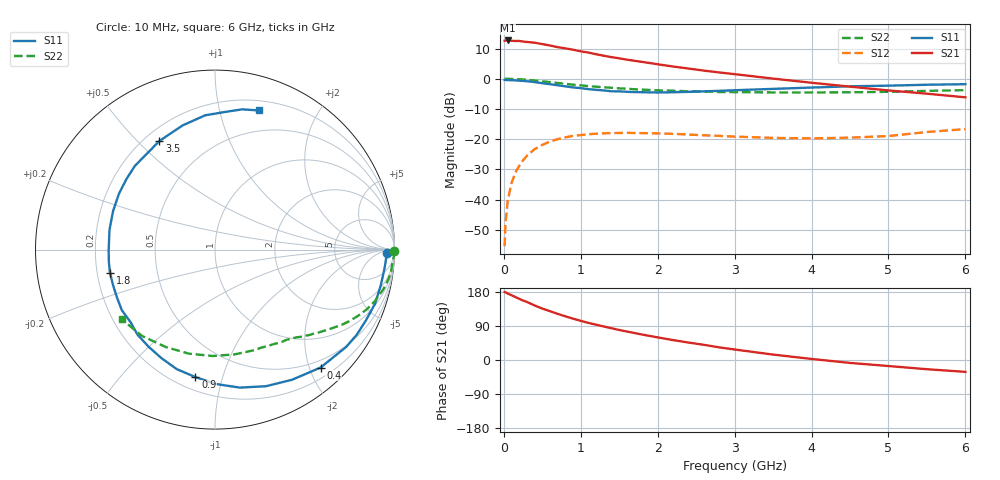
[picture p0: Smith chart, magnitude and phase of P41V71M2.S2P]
! SIEMENS Small Signal Semiconductors
! BFP182
! Si NPN RF Bipolar Junction Transistor in SOT143
! VCE = 1.75 V  IC = 1.2 mA
! Common Emitter S-Parameters:  March  1996
# GHz  S  MA  R  50
!  f  S11  S21  S12  S22
! GHz  MAG  ANG  MAG  ANG  MAG  ANG  MAG  ANG
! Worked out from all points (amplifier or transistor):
!   36 points, 10 MHz to 6 GHz, reference 50 ohm
!   highest |S21| = 12.7 dB at 50 MHz (marker M1)
!   |S21| within 3 dB of that: start of sweep to 884.8 MHz
!   unconditionally stable (mu >= 1): 2.497 GHz to end of sweep
!   at 250 MHz: K = 0.10, MSG = 19.6 dB, |S12| = -27.0 dB
!   at 1.4 GHz: K = 0.58, MSG = 12.6 dB, |S12| = -18.0 dB
!   at 6 GHz: K = 1.07, MAG = 3.6 dB, |S12| = -16.7 dB
!   S11 on the Smith chart (normalised r, x): 10 MHz: 37, -16; 400 MHz: 0.37, -2.18; 900 MHz: 0.28, -0.82; 1.8 GHz: 0.25, -0.10; 3.5 GHz: 0.26, +0.58; 6 GHz: 0.29, +1.32
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0.01  0.9558 -1.1  4.259 179.4  0.0017 88.1  0.9985 -0.4
0.02  0.9552 -2.6  4.273 178.8  0.0038 81.7  0.9999 -1.0
0.05  0.9505 -6.3  4.3 175.4  0.0096 89.3  0.9966 -2.3
0.1  0.9447 -12.2  4.251 170.9  0.0188 82.2  0.9905 -4.7
0.15  0.9413 -18.6  4.211 166.2  0.028 78.3  0.9889 -7.1
0.2  0.929 -25.0  4.221 161.4  0.0362 74.7  0.981 -9.4
0.4  0.8819 -48.2  3.947 143.9  0.0684 61.1  0.9365 -17.8
0.5  0.8426 -59.4  3.745 135.8  0.0805 54.5  0.9077 -21.6
0.6  0.8122 -69.6  3.55 128.7  0.0915 48.7  0.8785 -24.8
0.7  0.7813 -79.8  3.329 121.8  0.1002 43.6  0.8513 -27.7
0.8  0.7492 -89.4  3.183 115.2  0.1072 38.8  0.8252 -30.3
0.9  0.7189 -98.7  3.02 109.1  0.1134 34.2  0.7982 -32.7
1.1  0.674 -116.4  2.708 97.8  0.121 26.9  0.756 -36.8
1.3  0.641 -132.4  2.403 88.3  0.1252 20.5  0.7221 -40.4
1.5  0.6192 -147.0  2.178 79.2  0.1267 15.6  0.694 -43.7
1.8  0.5993 -167.7  1.899 67.0  0.1262 9.9  0.6605 -48.2
2.2  0.5981 169.4  1.593 52.5  0.1227 4.1  0.6337 -54.5
2.8  0.631 141.4  1.272 33.4  0.1135 0.1  0.6037 -65.0
3.5  0.6798 117.1  1.005 14.3  0.1051 0.6  0.594 -79.4
4.5  0.7502 94.2  0.74 -7.7  0.1061 8.5  0.5977 -104.1
5.5  0.7961 79.0  0.566 -24.3  0.1314 14.8  0.63 -130.3
6  0.8128 72.5  0.493 -31.3  0.147 13.2  0.648 -143.1
